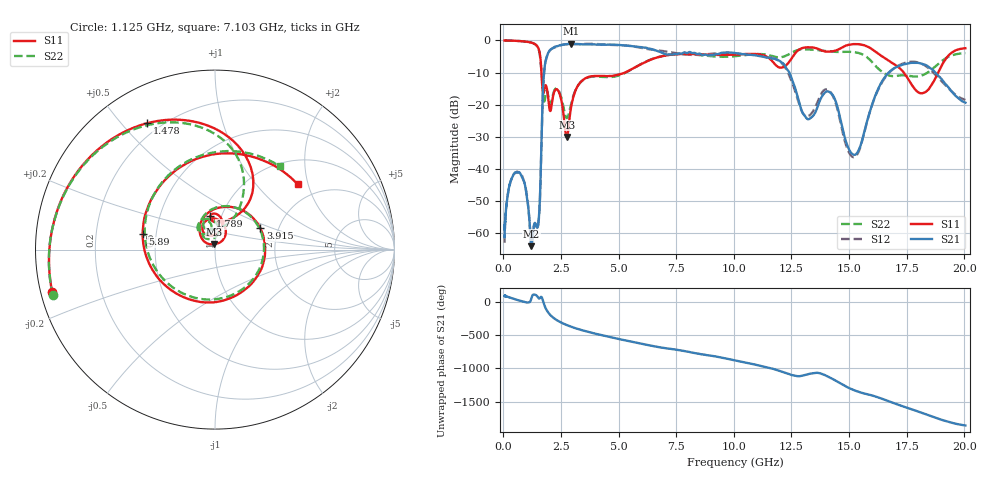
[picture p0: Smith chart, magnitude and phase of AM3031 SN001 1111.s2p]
# Hz S DB R 50
!freq MagS11 AngS11 MagS21 AngS21 MagS12 AngS12 MagS22 AngS22
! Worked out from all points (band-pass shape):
!   1601 points, 50 MHz to 20.05 GHz, reference 50 ohm
!   highest |S21| = -1.04 dB at 2.934 GHz (marker M1); lowest = -64.0 dB at 1.217 GHz (marker M2)
!   |S21| within 3 dB of the highest: 1.934 GHz to 6.94 GHz (5.006 GHz wide, 113 % of centre); 9.397 GHz to 10.15 GHz (756.4 MHz wide, 7.74 % of centre)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
!   lowest |S11| = -30.0 dB at 2.743 GHz (marker M3), VSWR 1.07, Z = 49.6 + j3.11 ohm
!   |S11| at or under -10 dB: 1.648 GHz to 5.276 GHz (3.628 GHz wide, 105 % of centre); 17.37 GHz to 18.87 GHz (1.495 GHz wide, 8.25 % of centre)
!   |S22| runs from -24.2 to 0.0 dB; largest |S21 - S12| = 0.068
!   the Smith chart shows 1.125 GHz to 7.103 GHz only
!   S11 on the Smith chart (normalised r, x): 1.125 GHz: 0.03, -0.13; 1.478 GHz: 0.15, +0.59; 1.789 GHz: 0.89, +0.34; 3.915 GHz: 1.61, +0.42; 5.89 GHz: 0.42, +0.09; 7.103 GHz: 1.54, +1.72
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5e7  -0.03 -7.3  -61.05 88.4  -62.93 78.9  -0.04 -7.1
1.35947e8  -0.06 -19.1  -50.76 83.2  -50.75 83.6  -0.05 -19.1
3.696318e8  -0.10 -51.4  -42.75 55.2  -42.62 55.7  -0.10 -52.0
1.005007e9  -0.42 -145.5  -48.07 -9.3  -47.59 -8.0  -0.41 -144.9
1.124547e9  -0.56 -165.4  -55.58 -5.0  -55.76 -7.2  -0.55 -164.4
1.216589e9  -0.72 178.0  -63.97 61.1  -63.61 61.0  -0.70 179.5
1.478245e9  -1.94 118.4  -58.15 78.0  -58.27 76.4  -1.98 120.4
1.789457e9  -14.45 98.0  -8.12 -61.5  -8.26 -61.6  -18.75 106.1
2.040165e9  -21.92 104.7  -2.88 160.6  -2.97 161.1  -19.95 118.1
2.722335e9  -29.84 85.4  -1.19 15.8  -1.22 16.2  -23.97 97.6
2.742808e9  -30.03 96.4  -1.19 12.8  -1.21 13.3  -24.14 103.0
2.934141e9  -20.85 140.9  -1.04 -12.6  -1.17 -12.2  -19.78 132.3
3.915228e9  -11.07 25.6  -1.22 -111.1  -1.07 -111.3  -11.24 28.4
5.889746e9  -7.69 167.7  -2.07 98.9  -2.20 98.5  -7.68 161.0
7.103038e9  -4.62 38.4  -4.40 22.0  -3.52 21.3  -4.61 52.0
7.401857e9  -4.36 10.3  -4.25 8.1  -3.91 3.7  -4.36 26.8
8.76102e9  -4.40 -108.3  -4.40 -75.7  -4.36 -72.6  -4.74 -92.9
1.056581e10  -4.22 84.1  -4.43 164.3  -4.38 165.2  -4.50 80.0
1.293477e10  -2.49 -100.9  -21.74 -31.2  -21.74 -22.8  -2.78 -94.8
1.51388e10  -1.21 97.3  -35.30 123.9  -36.19 126.6  -3.62 110.1
1.725979e10  -9.09 -54.5  -7.72 -119.9  -7.44 -116.6  -10.85 -82.8
2.005e10  -2.45 63.0  -19.36 -57.0  -18.54 -53.7  -3.98 73.9
